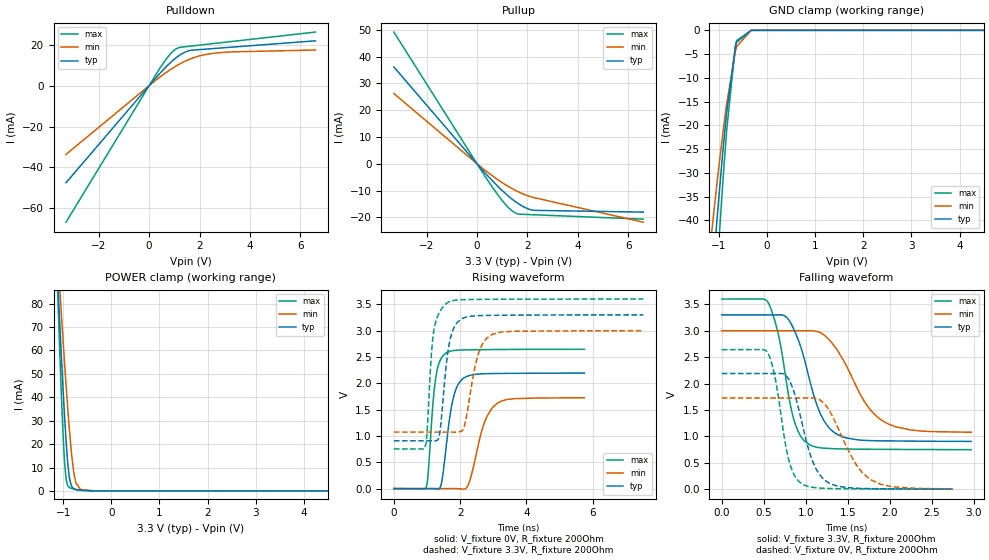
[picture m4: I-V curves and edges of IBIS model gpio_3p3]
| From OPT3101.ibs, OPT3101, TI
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|   gpio_3p3 Model
[Model]   gpio_3p3
Model_type   I/O
Polarity   Non-Inverting
Enable   Active-High
Vinl = 0.99
Vinh = 2.31
Vmeas = 1.65
Vref = 0
Cref = 2pF
Rref = 200
|   typ   min   max
|   (nom PVT)   (fast PVT)   (slow PVT)
C_comp   2.219e-12   1.984e-12   2.430e-12
[Model spec]
|subparameter
Vinl   0.99   0.90   1.08
Vinh   2.31   2.10   2.52
| Where nom  PVT is Nominal Process, 3.3V, 27C
|   Fast PVT is Strong Process,  3.6V, -40C
|   Slow PVT is Weak Process,   3V, 125C
[Voltage Range]   3.3   3   3.6
|Junction Temperature
[Temperature Range]   27   125   -40
[Pullup Reference]   3.3   3   3.6
[Pulldown Reference]   0   0   0
[Power Clamp Reference]   3.3   3   3.6
[GND Clamp Reference]   0   0   0
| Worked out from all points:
|   slope of the pulldown table from 0 to 0.495 V, typ, clamps not added: 71.8 ohm
|   slope of the pullup table from 0 to 0.495 V, typ, clamps not added: 95.4 ohm
|   POWER clamp passes 1 mA (typ) near -0.78 V on its own axis
|   falling waveform, V_fixture 3.3V, R_fixture 200Ohm: 20-80 % time 275ps typ, 410ps min, 200ps max; typ from 3.3 V to 0.905 V
|   rising waveform, V_fixture 0V, R_fixture 200Ohm: 20-80 % time 294ps typ, 443ps min, 204ps max; typ from 0 V to 2.19 V
|   rising waveform, V_fixture 3.3V, R_fixture 200Ohm: 20-80 % time 251ps typ, 366ps min, 190ps max; typ from 0.908 V to 3.3 V
|   falling waveform, V_fixture 0V, R_fixture 200Ohm: 20-80 % time 230ps typ, 339ps min, 168ps max; typ from 2.19 V to 0.003 V
[Pulldown]
|   Voltage   I(typ)   I(min)   I(max)
-3.3V     -47.49mA   -33.64mA   -66.79mA
307.2mV   4.367mA    3.067mA    6.17mA
762mV     10.28mA    7.183mA    14.35mA
1.031V    13.25mA    9.318mA    17.65mA
1.203V    14.84mA    10.55mA    18.67mA
1.441V    16.5mA     12.05mA    19.05mA
1.623V    17.24mA    13.03mA    19.31mA
2.043V    17.67mA    14.72mA    19.89mA
2.521V    18.12mA    15.77mA    20.55mA
3.29V     18.84mA    16.53mA    21.62mA
6.6V      21.94mA    17.43mA    26.2mA
[GND Clamp]
|   Voltage   I(typ)   I(min)   I(max)
-3.3V     -1.435A    -1.247A    -1.587A
-1.188V   -59.19mA   -46.31mA   -75.72mA
-1.093V   -46.61mA   -37.13mA   -59.51mA
-1.023V   -37.77mA   -30.66mA   -48.01mA
-1.021V   -37.55mA   -30.5mA    -47.72mA
-914.1mV  -25.09mA   -21.32mA   -31.35mA
-840mV    -17.39mA   -15.55mA   -21.19mA
-660mV    -3.71mA    -4.587mA   -3.526mA
-632.4mV  -2.514mA   -3.451mA   -2.169mA
-330mV    -1.062uA   -12.81uA   -96.75nA
6.6V      0A         0A         0A
[Pullup]
|   Voltage   I(typ)   I(min)   I(max)
-3.3V     36.16mA    26.24mA    49.2mA
361.2mV   -3.83mA    -2.739mA   -5.255mA
867.9mV   -8.806mA   -6.223mA   -12.12mA
1.063V    -10.56mA   -7.433mA   -14.45mA
1.384V    -13.14mA   -9.229mA   -17.52mA
1.65V     -14.96mA   -10.52mA   -18.79mA
2.043V    -16.9mA    -12.04mA   -18.96mA
2.247V    -17.4mA    -12.62mA   -19.04mA
6.6V      -18.06mA   -21.82mA   -20.7mA
[POWER Clamp]
|   Voltage   I(typ)   I(min)   I(max)
-3.3V     1.113A     867.8mA    1.544A
-1.129V   96.9mA     105.9mA    94.41mA
-1.102V   85.27mA    97.07mA    78.25mA
-1.068V   70.53mA    85.71mA    58.13mA
-999.6mV  42.66mA    63.62mA    23.06mA
-970.2mV  31.75mA    54.47mA    12.19mA
-940.5mV  21.81mA    45.53mA    5.456mA
-903mV    11.6mA     34.81mA    2.221mA
-834.9mV  2.433mA    17.82mA    1.123mA
-738mV    595.3uA    3.664mA    629.8uA
-636mV    257uA      540.1uA    255.4uA
6.6V      0A         0A         0A
[Ramp]
R_load = 200
|   typ   min   max
dV/dt_r   1.316/2.93202e-10   1.03695/4.42937e-10   1.5882/2.03924e-10
dV/dt_f   1.43855/2.75294e-10  1.15718/4.11829e-10   1.71235/2.00086e-10
[Falling Waveform]
V_fixture = 3.3V
V_fixture_min = 3V
V_fixture_max = 3.6V
R_fixture = 200Ohm
|   Time   V(typ)   V(min)   V(max)
0s        3.3V       3V         3.6V
550ps     3.3V       3V         3.541V
680ps     3.301V     3V         2.892V
860ps     3.023V     3V         1.313V
1.06ns    1.983V     3.001V     831.3mV
1.18ns    1.411V     2.961V     783.5mV
1.33ns    1.086V     2.735V     768.2mV
1.71ns    924.7mV    1.634V     757.3mV
1.92ns    916mV      1.291V     755.3mV
2.97ns    905.5mV    1.079V     749.2mV
[Rising Waveform]
V_fixture = 0V
V_fixture_min = 0V
V_fixture_max = 0V
R_fixture = 200Ohm
|   Time   V(typ)   V(min)   V(max)
0s        1.297nV    41.81nV    828.7pV
970ps     -19.32uV   33.83nV    16.48mV
1.27ns    -4.6mV     34.13nV    2.128V
1.43ns    83.91mV    34.82nV    2.474V
1.58ns    805.1mV    -47.5uV    2.578V
1.81ns    1.76V      531uV      2.623V
2.13ns    2.109V     -8.83mV    2.634V
2.76ns    2.182V     1.297V     2.64V
3.13ns    2.187V     1.624V     2.642V
5.75ns    2.194V     1.726V     2.646V
[Rising Waveform]
V_fixture = 3.3V
V_fixture_min = 3V
V_fixture_max = 3.6V
R_fixture = 200Ohm
|   Time   V(typ)   V(min)   V(max)
0s        907.9mV    1.073V     753.9mV
930ps     907.9mV    1.073V     762.9mV
990ps     907.9mV    1.073V     974.1mV
1.2ns     906.7mV    1.073V     2.974V
1.39ns    1.074V     1.073V     3.363V
1.63ns    2.592V     1.074V     3.535V
2.1ns     3.24V      1.137V     3.589V
2.56ns    3.285V     2.579V     3.593V
2.97ns    3.291V     2.931V     3.596V
7.53ns    3.3V       2.999V     3.6V
[Falling Waveform]
V_fixture = 0V
V_fixture_min = 0V
V_fixture_max = 0V
R_fixture = 200Ohm
|   Time   V(typ)   V(min)   V(max)
0s        2.191V     1.727V     2.643V
560ps     2.19V      1.727V     2.546V
640ps     2.191V     1.727V     2.075V
800ps     2.075V     1.727V     544.6mV
950ps     1.293V     1.727V     107.1mV
1.12ns    394.5mV    1.718V     29.04mV
1.3ns     101.6mV    1.439V     13.51mV
1.6ns     19.95mV    468.5mV    7.198mV
1.77ns    11.07mV    185mV      5.807mV
2.75ns    3.203mV    5.813mV    1.421mV
